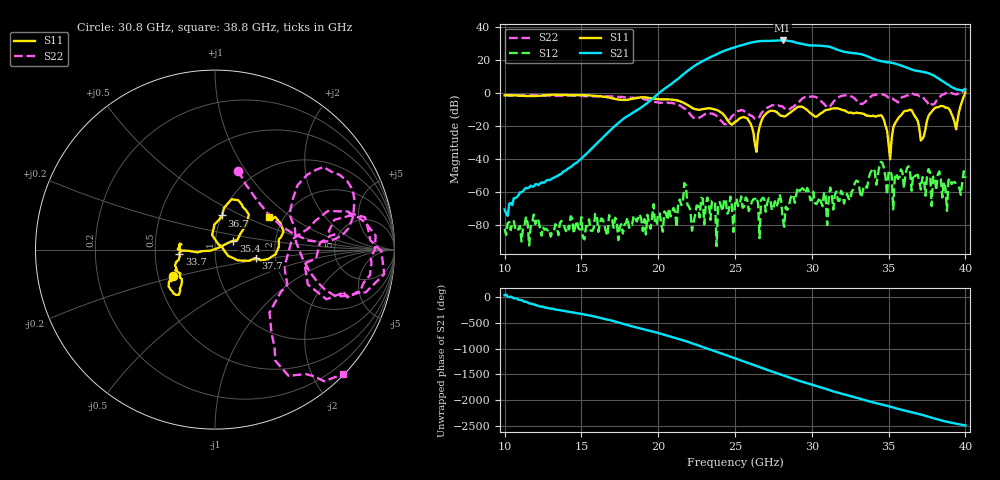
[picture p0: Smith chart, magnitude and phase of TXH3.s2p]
!Keysight Technologies,M9808A,MY58100618,A.14.70.03
!Date: Monday, February 27, 2023 13:37:00
!Correction: S11(C  2-Port  )
!S21(C  2-Port  )
!S12(C  2-Port  )
!S22(C  2-Port  )
!S2P File: Measurements: S11, S21, S12, S22:
# Hz S  RI  R 50
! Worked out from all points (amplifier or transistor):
!   301 points, 10 GHz to 40 GHz, reference 50 ohm
!   highest |S21| = 31.6 dB at 28.1 GHz (marker M1)
!   |S21| within 3 dB of that: 25.39 GHz to 29.91 GHz (4.516 GHz wide, 16.3 % of centre)
!   unconditionally stable (mu >= 1): start of sweep to 39.75 GHz
!   at 15 GHz: K = 30436.70, MAG = -30.1 dB, |S12| = -75.4 dB
!   at 25 GHz: K = 46.02, MAG = 27.9 dB, |S12| = -67.5 dB
!   at 40 GHz: K = 2.30, MSG = 26.8 dB, |S12| = -51.6 dB
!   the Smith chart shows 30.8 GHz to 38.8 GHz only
!   S11 on the Smith chart (normalised r, x): 30.8 GHz: 0.60, -0.19; 33.7 GHz: 0.67, -0.03; 35.4 GHz: 1.22, +0.12; 36.7 GHz: 1.00, +0.40; 37.7 GHz: 1.58, -0.16; 38.8 GHz: 1.68, +0.68
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1e10  0.7544 0.3339  0.000222 0.000189  7.27e-05 -2.21e-05  0.0297 0.8537
1.5e10  0.6124 -0.582  0.00823 0.00587  -0.000138 9.85e-05  0.737 0.305
2e10  -0.1607 -0.6122  0.8516 0.3672  -0.000169 -0.000149  0.2588 -0.4307
2.34e10  -0.3369 -0.0119  6.228 10.12  -0.000106 9.19e-05  -0.1016 -0.2109
2.42e10  -0.2281 -0.0344  16.1 -7.503  2.95e-06 -0.000257  -0.0842 -0.0931
2.5e10  -0.0579 0.1158  -8.348 -22.37  8.44e-06 -0.000424  -0.2268 0.0402
2.58e10  -0.0568 0.1547  -29.7 7.656  -0.000441 -0.000366  -0.2509 0.0222
2.66e10  0.0566 -0.0717  7.589 35.45  2.47e-05 3.03e-05  -0.0527 0.1777
2.74e10  0.2499 -0.1345  37.09 -4.278  -8.97e-05 -0.000257  -0.0505 0.413
2.81e10  0.1282 -0.151  7.027 -37.5  -8.78e-05 -0.000142  -0.06 0.375
2.89e10  -0.0193 -0.3199  -32.07 -9.877  -0.000411 -0.000208  0.2959 0.2893
3e10  0.0107 -0.2217  -3.941 26.64  6.64e-05 0.000555  0.2924 0.7071
3.08e10  -0.235 -0.1472  23.4 10.91  -0.000327 0.000919  0.13 0.4394
3.19e10  -0.1977 -0.2399  4.443 -18  0.000519 0.000934  0.7703 0.1836
3.29e10  -0.2218 -0.1143  -14.24 -6.408  -0.000405 0.00214  0.46 0.3595
3.37e10  -0.1992 -0.0227  -8.444 8.827  -0.000205 0.00251  0.6128 -0.2229
3.5e10  -0.0268 -0.00649  6.729 4.882  -0.00269 -0.00298  0.6653 0.1661
3.54e10  0.1023 0.0488  7.647 0.4955  -0.00241 -0.000943  0.5837 0.035
3.67e10  0.0397 0.1905  -0.3987 -4.684  0.000465 0.00289  0.8657 0.0522
3.77e10  0.2273 -0.047  -3.712 -0.2059  -0.00325 -0.00228  0.3858 -0.0997
3.88e10  0.2987 0.179  -0.1125 1.809  0.000263 5.2e-06  0.7107 -0.6951
4e10  0.4463 -0.9031  1.158 0.4654  0.00259 -0.000442  1.236 -0.6069
